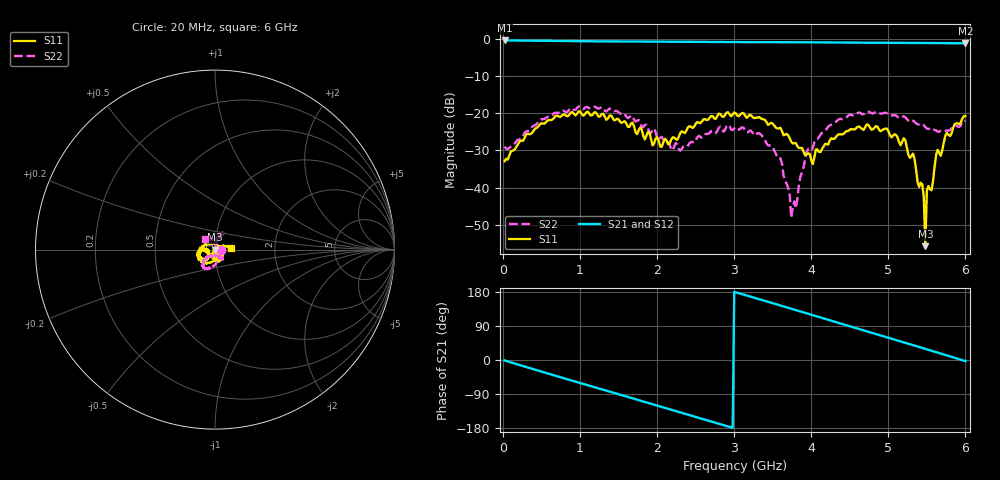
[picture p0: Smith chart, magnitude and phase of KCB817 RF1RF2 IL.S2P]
!Agilent Technologies,E5071B,JP1KK00126,A.08.11
!Date: Mon Apr 22 13:19:14 2013
!Data & Calibration Information:
!Freq	S11:SOLT2(ON)	S21:SOLT2(ON)	S12:SOLT2(ON)	S22:SOLT2(ON)
# Hz S dB R 50
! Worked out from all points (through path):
!   300 points, 20 MHz to 6 GHz, reference 50 ohm
!   highest |S21| = -0.38 dB at 20 MHz (marker M1); lowest = -1.2 dB at 6 GHz (marker M2)
!   group delay of S21, straight-line fit = 167 ps
!   lowest |S11| = -55.8 dB at 5.48 GHz (marker M3), VSWR 1.00, Z = 50.2 + j0.0253 ohm
!   |S11| at or under -10 dB: start of sweep to end of sweep
!   |S22| runs from -48.1 to -18.1 dB; largest |S21 - S12| = 0.0051
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2e7  -32.89 -12.7  -0.38 -1.2  -0.35 -1.4  -28.94 -7.2
5e8  -22.67 -104.6  -0.47 -30.7  -0.46 -30.8  -21.57 -89.2
1.02e9  -20.11 -145.6  -0.58 -61.9  -0.57 -62.0  -18.75 -116.6
2.02e9  -27.41 -152.2  -0.70 -121.5  -0.69 -121.6  -27.17 -123.4
2.3e9  -25.26 -135.4  -0.73 -138.2  -0.73 -138.5  -30.05 -87.0
3.02e9  -20.02 -156.0  -0.82 178.7  -0.80 178.5  -23.74 -54.3
3.6e9  -23.86 152.9  -0.84 143.8  -0.82 143.7  -32.12 -68.9
3.72e9  -26.66 138.7  -0.84 136.5  -0.83 136.4  -41.95 -79.6
3.74e9  -27.62 134.0  -0.85 135.3  -0.83 135.2  -48.07 -63.5
3.94e9  -31.08 68.5  -0.87 123.2  -0.85 123.0  -30.45 82.7
4.02e9  -33.67 49.1  -0.88 118.3  -0.85 118.1  -29.24 86.7
4.52e9  -24.22 -52.7  -0.95 87.8  -0.95 87.8  -20.46 74.2
5.02e9  -25.76 -92.4  -1.01 57.6  -1.01 57.4  -20.35 63.9
5.32e9  -30.83 -126.3  -1.05 39.2  -1.04 39.0  -21.94 66.2
5.38e9  -38.58 -125.6  -1.05 35.5  -1.04 35.4  -22.99 70.2
5.44e9  -39.10 -144.8  -1.06 31.8  -1.05 31.7  -22.98 71.7
5.46e9  -42.44 -137.1  -1.06 30.6  -1.05 30.5  -23.20 73.3
5.48e9  -55.76 8.9  -1.06 29.4  -1.05 29.3  -23.68 77.0
5.5e9  -40.74 38.8  -1.06 28.1  -1.05 28.1  -24.09 81.3
5.56e9  -40.71 61.5  -1.08 24.4  -1.06 24.3  -23.95 81.6
5.64e9  -29.83 35.0  -1.08 19.5  -1.07 19.4  -24.92 96.5
6e9  -20.70 6.0  -1.15 -2.8  -1.14 -2.9  -22.03 132.8
